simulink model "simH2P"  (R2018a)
settings: Solver=ode15s  StartTime=0.0  StopTime=tsim  MaxStep=1  RelTol=1e-3
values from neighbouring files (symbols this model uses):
  Kalg = [zeros(nz,nx),eye(nz)]    [runH2Psim.m]
  KcA = 1/kTA*tauTA/(taucTA+thetaTA)    (= -0.000770712909441)    [runH2Psim.m]    (also in H2P_Turbine_driven.m = ctrl(5); runTD.m; H2P_Boiler_driven.m = ctrl(5); runBD.m)
  KcD = 1/kD*1/(taucD+thetaD)    (= 0.103092783505)    [runH2Psim.m]    (also in H2P_Turbine_driven.m = ctrl(2); runTD.m; H2P_Boiler_driven.m = ctrl(2); runBD.m = 0.00343642611684)
  KcTG = 1/kTG*tauTG/(taucTG+thetaTG)    (= 0.0511927920549)    [runH2Psim.m]    (also in H2P_Turbine_driven.m = ctrl(8); runTD.m; H2P_Boiler_driven.m = ctrl(8); runBD.m)
  Kdyn = [eye(nx),zeros(nx,nz)]    [runH2Psim.m]
  KMD = zeros(nv,1); KMD(4) = 1    [runH2Psim.m]
  KPm = zeros(nv,1); KPm(12)= 1    [runH2Psim.m]
  KTA = zeros(nv,1); KTA(7) = 1    [runH2Psim.m]
  KTG = zeros(nv,1); KTG(8) = 1    [runH2Psim.m]
  mA0 = mA    [runH2Psim.m]    (also in H2P_Turbine_driven.m = ctrl(4); H2P_Boiler_driven.m = ctrl(4); H2P_Floating_pressure.m = ctrl(4); H2P_VPC.m = ctrl(4))
  MDsp = MD0    (= 3000)    [runH2Psim.m]    (also in H2P_Turbine_driven.m = u(2); runTD.m; H2P_Boiler_driven.m = u(2); runBD.m)
  mG0 = mG    [runH2Psim.m]    (also in H2P_Turbine_driven.m = ctrl(10); H2P_Boiler_driven.m = ctrl(10); H2P_Floating_pressure.m = ctrl(10); H2P_VPC.m = ctrl(13))
  mP0 = mA+m    [runH2Psim.m]    (also in H2P_Turbine_driven.m = ctrl(1); H2P_Boiler_driven.m = ctrl(1); H2P_Floating_pressure.m = ctrl(1); H2P_VPC.m = ctrl(1))
  np = length(param)    [runH2Psim.m]    (also in Main.m = size(p,2); Main_OL.m = size(p,2); runTestCalcBlk.m = size(p,2); runTransf.m = size(p,2))
  nu = length(u0)    [runH2Psim.m]    (also in Main.m = 1; Main_OL.m = 1; runTestCalcBlk.m = 1; runTransf.m = 1)
  nv = length(v0)    [runH2Psim.m]
  param = [Tref;TrefB;dHvap;cpg;cpW;cpSt;R;Mwt;          T0;TG0;ME;pC;          UAE; UAD; UASh; CvD; Kv; VSh; phid;          Pm0; w0; M0; D0; PL; nx]    [runH2Psim.m]    (also in runTD.m = [Tref;TrefB;dHvap;cpg;cpW;cpSt;R;Mwt;     T0;TG0;ME;pC;     ; runBD.m; runFP.m; runFPV2.m)
  Pm0 = param(20)    [H2P.m]    (also in runH2Psim.m = W0; H2P_Turbine_driven.m; runTD.m = W0; H2P_Boiler_driven.m)
  Pmsp = Pm0*0.9    [runH2Psim.m]    (also in H2P_Turbine_driven.m = u(1); H2P_Boiler_driven.m = u(1); runBD.m = Pm0*1.1; H2P_Floating_pressure.m = u(1))
  TAsp = 802    [runH2Psim.m]    (also in H2P_Turbine_driven.m = u(4); runTD.m; H2P_Boiler_driven.m = u(4); runBD.m)
  tauIA = min(tauTA,4*(taucTA+thetaTA))    [runH2Psim.m]    (also in H2P_Turbine_driven.m = ctrl(6); runTD.m; H2P_Boiler_driven.m = ctrl(6); runBD.m)
  tauID = 4*(taucD+thetaD)    (= 40)    [runH2Psim.m]    (also in H2P_Turbine_driven.m = ctrl(3); runTD.m; H2P_Boiler_driven.m = ctrl(3); runBD.m = 1200)
  tauITG = min(tauTG,4*(taucTG+thetaTG))    [runH2Psim.m]    (also in H2P_Turbine_driven.m = ctrl(9); runTD.m; H2P_Boiler_driven.m = ctrl(9); H2P_Floating_pressure.m = ctrl(9))
  tauIzPm = min(tauzPm,4*(tauczPm+thetazPm))    [runH2Psim.m]    (also in H2P_VPC.m = ctrl(12); runVPC.m)
  TGsp = 423    [runH2Psim.m]    (also in runTD.m; runBD.m; runFP.m; runFPV2.m)
  u0 = [mG0;zV0;mP0;mB0;mA0]    [runH2Psim.m]    (also in calcblock.m = p(2); testfun.m = 5; u_function.m = 5; calcblock3.m = p(2))
  x0 = [TE0;TD0;TSh0;MD0; MSh0;w0;TA0]    [runH2Psim.m]    (also in runTD.m = [TE0;TD0;TSh0;MD0; MSh0;w0;TA0;0;0;0;0;0;0;0;0;0]; runBD.m = [TE0;TD0;TSh0;MD0; MSh0;w0;TA0;0;0;0;0;0;0;0;0;0]; runFP.m = [TE0;TD0;TSh0;MD0; MSh0;w0;TA0;0;0;0;0;0;0;0]; runFPV2.m = [TE0;TD0;TSh0;MD0; MSh0;w0;TA0;0;0;0;0;0;0;0])
  z0 = [TGE0;TGD;TGSh;pT; Pm0]    [runH2Psim.m]    (also in runTD.m = [TGE0;TGD;TGSh;pT; Pm0;mG;zV]; runBD.m = [TGE0;TGD;TGSh;pT; Pm0;mG;zV]; runFP.m = [TGE0;TGD;TGSh;pT; Pm0;mG;zV]; runFPV2.m = [TGE0;TGD;TGSh;pT; Pm0;mG;zV])
  zV0 = 0.9    [runH2Psim.m]    (also in H2P_Turbine_driven.m = ctrl(13); H2P_Boiler_driven.m = ctrl(13); H2P_VPC.m = ctrl(10); H2P_2_controllers.m = ctrl(13))
undefined symbols (not defined in the file or in its folder): H2P

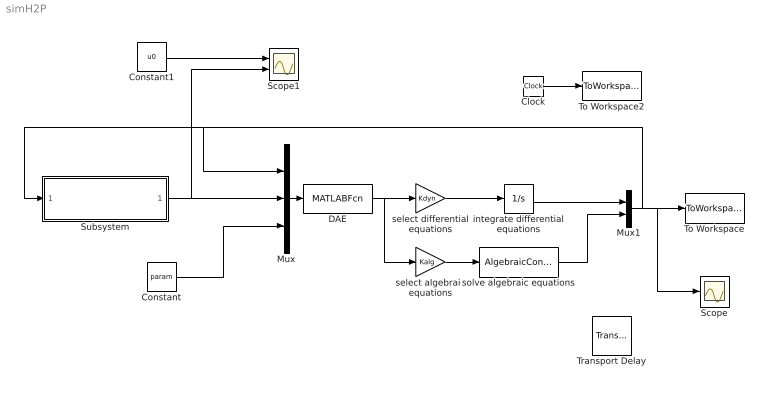
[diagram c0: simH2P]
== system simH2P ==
  Clock : Clock
  Constant : Constant  Value=param
  Constant1 : Constant  Value=u0
  DAE : MATLABFcn  MATLABFcn=H2P(u(1:nv), u(nv+1:nv+nu), u(nv+nu+1:nv+nu+np))  OutputDimensions=12
  Mux : Mux  Inputs=3
  Mux1 : Mux  Inputs=2
  Scope : Scope
  Scope1 : Scope  NumInputPorts=2
  Subsystem : Subsystem
  To Workspace : ToWorkspace  VariableName=v  SampleTime=-1
  To Workspace2 : ToWorkspace  VariableName=t  SampleTime=-1
  Transport Delay : TransportDelay  DelayTime=0  InitialOutput=z0
  integrate differential equations : Integrator  InitialCondition=x0
  select algebraic equations : Gain  Gain=Kalg  Multiplication=Matrix(K*u)
  select differential equations : Gain  Gain=Kdyn  Multiplication=Matrix(K*u)
  solve algebraic equations : AlgebraicConstraint  Solver=Trust region  InitialGuess=z0
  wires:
  integrate differential equations/1 -> Mux1/1
  select differential equations/1 -> integrate differential equations/1
  select algebraic equations/1 -> solve algebraic equations/1
  Mux/1 -> DAE/1
  Clock/1 -> To Workspace2/1
  Mux1/1 -> Scope/1, To Workspace/1, Subsystem/1(Outputs), Mux/1
  DAE/1 -> select algebraic equations/1, select differential equations/1
  Subsystem/1("inputs ") -> Scope1/2, Mux/2
  Constant/1 -> Mux/3
  Constant1/1 -> Scope1/1
  solve algebraic equations/1 -> Mux1/2
  Transport Delay/1 -> ?

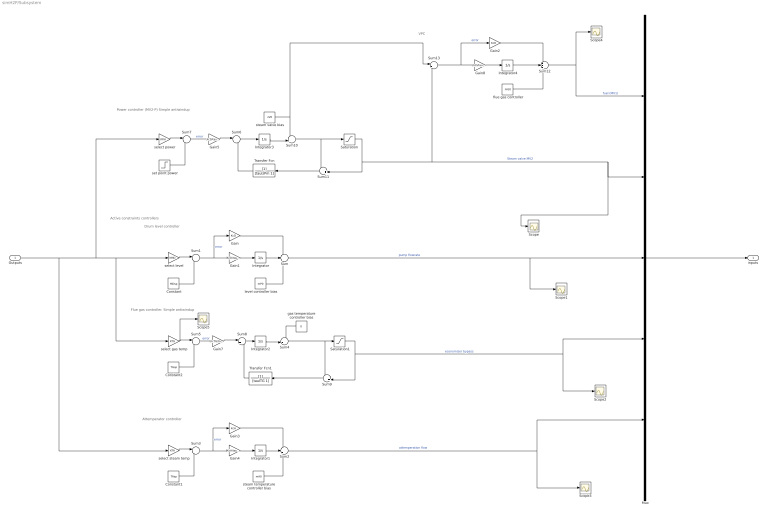
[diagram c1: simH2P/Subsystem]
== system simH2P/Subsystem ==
  note: Active constraints controllers
  note: Drum level controller
  note: Attemperator controller
  note: Flue gas controller. Simple antiwindup
  note: Power controller (MV2-P) Simple antiwindup
  note: VPC
  Outputs : Inport
  Constant : Constant  Value=MDsp
  Constant1 : Constant  Value=TAsp
  Constant2 : Constant  Value=TGsp
  Gain : Gain  Gain=KcD
  Gain1 : Gain  Gain=KcD/tauID  Multiplication=Matrix(K*u)
  Gain2 : Gain  Gain=KcD  Multiplication=Matrix(K*u)
  Gain3 : Gain  Gain=KcA
  Gain4 : Gain  Gain=KcA/tauIA  Multiplication=Matrix(K*u)
  Gain5 : Gain  Gain=KcD/tauID  Multiplication=Matrix(K*u)
  Gain7 : Gain  Gain=KcTG/tauITG  Multiplication=Matrix(K*u)
  Gain8 : Gain  Gain=KcD/tauID  Multiplication=Matrix(K*u)
  Integrator{,1..4} (5 alike) : Integrator
  Mux : Mux  Inputs=5
  Saturation : Saturate  UpperLimit=1  LowerLimit=0
  Saturation1 : Saturate  UpperLimit=inf  LowerLimit=0
  Scope{,1..5} (6 alike) : Scope
  Sum : Sum  Inputs=+++
  Sum{1,3,5,7} (4 alike) : Sum  Inputs=|-+
  Sum10 : Sum  Inputs=++|
  Sum11 : Sum  Inputs=-+|
  Sum12 : Sum  Inputs=+++
  Sum13 : Sum  Inputs=|+-
  Sum2 : Sum  Inputs=+++
  Sum4 : Sum  Inputs=++|
  Sum6 : Sum  Inputs=|++
  Sum8 : Sum  Inputs=|++
  Sum9 : Sum  Inputs=-+|
  Transfer Fcn : TransferFcn  Denominator=[tauIzPm 1]
  Transfer Fcn1 : TransferFcn  Denominator=[tauITG 1]
  flue gas controller : Constant  Value=mG0
  gas temperature controller bias : Constant  Value=0
  level controller bias : Constant  Value=mP0
  select gas temp : Gain  Gain=KTG  Multiplication=Matrix(u*K)
  select steam temp : Gain  Gain=KTA  Multiplication=Matrix(u*K)
  select level : Gain  Gain=KMD  Multiplication=Matrix(u*K)
  select power : Gain  Gain=KPm  Multiplication=Matrix(u*K)
  set point power : Step  Time=50  Before=Pm0  After=Pmsp  SampleTime=0
  steam temperature controller bias : Constant  Value=mA0
  steam valve bias : Constant  Value=zV0
  "inputs " : Outport
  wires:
  Mux/1 -> "inputs "/1
  Gain1/1 -> Integrator/1
  Integrator/1 -> Sum/2
  Gain/1 -> Sum/1
  Sum/1 -> Scope1/1, Mux/3  "pump flowrate"
  Sum1/1 -> Gain/1, Gain1/1  "error"
  Constant/1 -> Sum1/2
  select level/1 -> Sum1/1
  Constant1/1 -> Sum3/2
  Integrator1/1 -> Sum2/2
  Sum3/1 -> Gain3/1, Gain4/1  "error"
  Gain3/1 -> Sum2/1
  Gain4/1 -> Integrator1/1
  Sum2/1 -> Scope3/1, Mux/5  "attemperation flow"
  select steam temp/1 -> Sum3/1
  Constant2/1 -> Sum5/2
  Sum5/1 -> Gain7/1  "error"
  Gain7/1 -> Sum8/1
  Sum4/1 -> Saturation1/1, Sum9/1
  select gas temp/1 -> Scope5/1, Sum5/1
  Outputs/1 -> select level/1, select gas temp/1, select power/1, select steam temp/1
  Sum7/1 -> Gain5/1  "error"
  select power/1 -> Sum7/1
  Gain5/1 -> Sum6/1
  set point power/1 -> Sum7/2
  Integrator3/1 -> Sum10/2
  Sum6/1 -> Integrator3/1
  Transfer Fcn/1 -> Sum6/2
  level controller bias/1 -> Sum/3
  gas temperature controller bias/1 -> Sum4/1
  steam temperature controller bias/1 -> Sum2/3
  Saturation1/1 -> Sum9/2, Scope2/1, Mux/4  "economizer bypass"
  Integrator2/1 -> Sum4/2
  Sum8/1 -> Integrator2/1
  Transfer Fcn1/1 -> Sum8/2
  Sum9/1 -> Transfer Fcn1/1
  Sum10/1 -> Saturation/1, Sum11/1
  steam valve bias/1 -> Sum13/1, Sum10/1
  Sum11/1 -> Transfer Fcn/1
  flue gas controller/1 -> Sum12/3
  Sum12/1 -> Scope4/1, Mux/1  "fuel (MV1)"
  Sum13/1 -> Gain2/1, Gain8/1  "error"
  Saturation/1 -> Sum11/2, Sum13/2, Scope/1, Mux/2  "Steam valve MV2"
  Gain8/1 -> Integrator4/1
  Gain2/1 -> Sum12/1
  Integrator4/1 -> Sum12/2
